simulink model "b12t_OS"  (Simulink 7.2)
settings: Solver=ode3  SolverMode=SingleTasking  StartTime=0.0  StopTime=0.2  FixedStep=10e-6  MaxStep=1e-5  RelTol=1e-4  AbsTol=1e-4

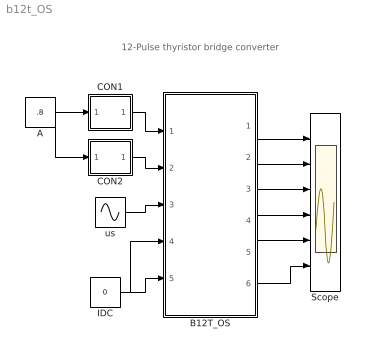
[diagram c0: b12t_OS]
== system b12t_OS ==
  note: 12-Pulse thyristor bridge converter
  A : Constant  Value=.8
  B12T_OS : Subsystem  mask{LS=1e-4, LT1=1e-4, LT2=1e-4, LD=1e-3, ILD0=200, C=5e-3, VC0=500, RL=2}
      mask prompts: LS "source Inductance"; LT1 "TYY leakage Inductance"; LT2 "TYD leakage Inductance"; LD "DC Inductance"; ILD0 "Initial Current ILD0"; C "Load Capacitance"; VC0 "Initial Cap Voltage"; RL "Load Resistance"
      mask help: 12-Pulse Thyristor Bridge Converter Input Vector u: u[0]= B6T1_H1.gate u[1]= B6T1_H2.gate u[2]= B6T1_H3.gate u[3]= B6T1_H4.gate u[4]= B6T1_H5.gate u[5]= B6T1_H6.gate u[6]= B6T2_H1.gate u[7]= B6T2_H2.gate u[8]= B6T2_H3.gate u[9]= B6T2_H4.gate u[10]= B6T2_H5.gate u[11]= B6T2_H6.gate u[12]= Vs1.v u[13]= Vs2.v u[14]= Vs3.v u[15]= IDC1.i u[16]= IDC1.i Output Vector y: y[0]= B6T1_T11.I y[1]= B6T1_T11.V y[2]= B6T2_T11.I y[3]= B6T2_T11.V y[4]= Ls1.I y[5]= Ls2.I y[6]= Ls3.I y[7]= Ld1.I y[8]= Ld2.I y[6]= VDC.V y[9]= VC1.V y[10]= VC2.V Parameter Vector p: p[0]= Ls.L p[1]= TYY_LT.L p[2]= TYD_LT.L p[3]= Ld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
  CON1 : Subsystem  mask(B6THY-Con){F=50, PH=60, TD=2e-3}
      mask prompts: F "Frequency"; PH "Phase Angle (Degree)"; TD "Puls Duration"
      mask help: Control of one Thyristor in a line commutated Converter circuit
      mask init:
      | x=0:pi/20:2*pi;
      | y=cos(x);
  CON2 : Subsystem  mask(B6THY-Con){F=50, PH=-150+60, TD=2e-3}
      mask prompts: F "Frequency"; PH "Phase Angle (Degree)"; TD "Puls Duration"
      mask help: Control of one Thyristor in a line commutated Converter circuit
      mask init:
      | x=0:pi/20:2*pi;
      | y=cos(x);
  IDC : Constant  Value=0
  Scope : Scope  NumInputPorts=6
  us : Sin  Amplitude=230*sqrt(2)  Frequency=2*pi*50  Phase="[0,  -2*pi/3,  -4*pi/3]"  SampleTime=0
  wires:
  A/1 -> CON1/1(In1), CON2/1(In1)
  CON1/1(Out1) -> B12T_OS/1(SWs)
  us/1 -> B12T_OS/3(vS)
  CON2/1(Out1) -> B12T_OS/2(SWs1)
  B12T_OS/1(i1T1;v1T!) -> Scope/1
  B12T_OS/2(i2T1,i2T1) -> Scope/2
  B12T_OS/3("iL1, iL2, iL3") -> Scope/3
  IDC/1 -> B12T_OS/4(iDC1), B12T_OS/5(iDC2)
  B12T_OS/4(iDC1,iDC2) -> Scope/4
  B12T_OS/5(vDC1,vDC1) -> Scope/5
  B12T_OS/6(vC1,vC2) -> Scope/6

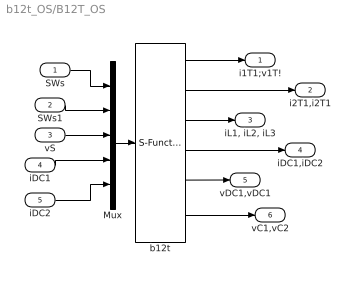
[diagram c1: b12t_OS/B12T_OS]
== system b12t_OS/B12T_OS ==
  SWs : Inport  OutDataType=sfix(16)  OutScaling=2^0
  SWs1 : Inport  Port=2  OutDataType=sfix(16)  OutScaling=2^0
  vS : Inport  Port=3  OutDataType=sfix(16)  OutScaling=2^0
  iDC1 : Inport  Port=4  OutDataType=sfix(16)  OutScaling=2^0
  iDC2 : Inport  Port=5  OutDataType=sfix(16)  OutScaling=2^0
  Mux : Mux  Inputs="[6   6   3  1  1]"
  b12t : S-Function  FunctionName=s_b12t_OS  Parameters="[LS  LT1 LT2  LD ILD0  C  VC0 RL]"  EnableBusSupport=off
  i1T1;v1T! : Outport  OutDataType=sfix(16)  OutScaling=2^0
  i2T1,i2T1 : Outport  Port=2  OutDataType=sfix(16)  OutScaling=2^0
  "iL1, iL2, iL3" : Outport  Port=3  OutDataType=sfix(16)  OutScaling=2^0
  iDC1,iDC2 : Outport  Port=4  OutDataType=sfix(16)  OutScaling=2^0
  vDC1,vDC1 : Outport  Port=5  OutDataType=sfix(16)  OutScaling=2^0
  vC1,vC2 : Outport  Port=6  OutDataType=sfix(16)  OutScaling=2^0
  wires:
  Mux/1 -> b12t/1
  iDC1/1 -> Mux/4
  b12t/2 -> i2T1,i2T1/1
  b12t/1 -> i1T1;v1T!/1
  vS/1 -> Mux/3
  SWs/1 -> Mux/1
  SWs1/1 -> Mux/2
  iDC2/1 -> Mux/5
  b12t/3 -> "iL1, iL2, iL3"/1
  b12t/4 -> iDC1,iDC2/1
  b12t/5 -> vDC1,vDC1/1
  b12t/6 -> vC1,vC2/1

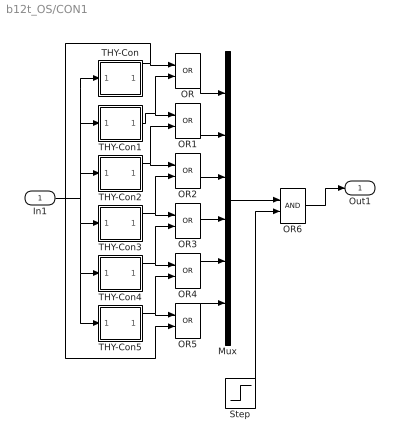
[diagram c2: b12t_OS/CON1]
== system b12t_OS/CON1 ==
  In1 : Inport
  Mux : Mux  Inputs=6
  OR{,1..5} (6 alike) : Logic  Operator=OR
  OR6 : Logic
  Step : Step  Time=1e-4  SampleTime=0
  THY-Con : Subsystem  mask(THY-Con){F=F, PH=PH, TD=TD}
      mask prompts: F "Frequency"; PH "Phase Angle (Degree)"; TD "Puls Duration"
      mask init:
      | x=0:pi/20:2*pi;
      | y=cos(x);
  THY-Con1 : Subsystem  mask(THY-Con){F=F, PH=PH-60, TD=TD}
      mask prompts: F "Frequency"; PH "Phase Angle (Degree)"; TD "Puls Duration"
      mask init:
      | x=0:pi/20:2*pi;
      | y=cos(x);
  THY-Con2 : Subsystem  mask(THY-Con){F=F, PH=PH-120, TD=TD}
      mask prompts: F "Frequency"; PH "Phase Angle (Degree)"; TD "Puls Duration"
      mask init:
      | x=0:pi/20:2*pi;
      | y=cos(x);
  THY-Con3 : Subsystem  mask(THY-Con){F=F, PH=PH-180, TD=TD}
      mask prompts: F "Frequency"; PH "Phase Angle (Degree)"; TD "Puls Duration"
      mask init:
      | x=0:pi/20:2*pi;
      | y=cos(x);
  THY-Con4 : Subsystem  mask(THY-Con){F=F, PH=PH-240, TD=TD}
      mask prompts: F "Frequency"; PH "Phase Angle (Degree)"; TD "Puls Duration"
      mask init:
      | x=0:pi/20:2*pi;
      | y=cos(x);
  THY-Con5 : Subsystem  mask(THY-Con){F=F, PH=PH-300, TD=TD}
      mask prompts: F "Frequency"; PH "Phase Angle (Degree)"; TD "Puls Duration"
      mask init:
      | x=0:pi/20:2*pi;
      | y=cos(x);
  Out1 : Outport
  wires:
  Step/1 -> OR6/2
  Mux/1 -> OR6/1
  In1/1 -> THY-Con/1(In1), THY-Con1/1(In1), THY-Con2/1(In1), THY-Con3/1(In1), THY-Con4/1(In1), THY-Con5/1(In1)
  THY-Con1/1(Out1) -> OR1/1, OR/2
  THY-Con2/1(Out1) -> OR2/1, OR1/2
  THY-Con3/1(Out1) -> OR3/1, OR2/2
  THY-Con4/1(Out1) -> OR4/1, OR3/2
  THY-Con5/1(Out1) -> OR5/1, OR4/2
  THY-Con/1(Out1) -> OR/1, OR5/2
  OR/1 -> Mux/1
  OR1/1 -> Mux/2
  OR2/1 -> Mux/3
  OR3/1 -> Mux/4
  OR4/1 -> Mux/5
  OR5/1 -> Mux/6
  OR6/1 -> Out1/1

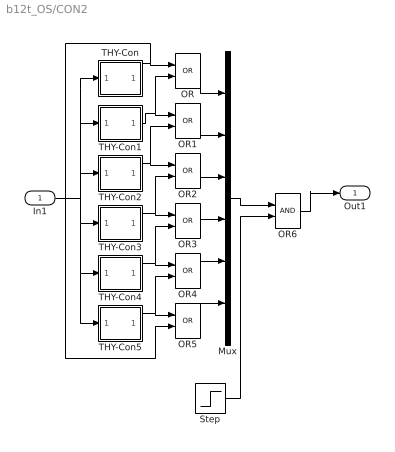
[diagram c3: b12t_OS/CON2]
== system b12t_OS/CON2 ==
  In1 : Inport
  Mux : Mux  Inputs=6
  OR{,1..5} (6 alike) : Logic  Operator=OR
  OR6 : Logic
  Step : Step  Time=1e-4  SampleTime=0
  THY-Con : Subsystem  mask(THY-Con){F=F, PH=PH, TD=TD}
      mask prompts: F "Frequency"; PH "Phase Angle (Degree)"; TD "Puls Duration"
      mask init:
      | x=0:pi/20:2*pi;
      | y=cos(x);
  THY-Con1 : Subsystem  mask(THY-Con){F=F, PH=PH-60, TD=TD}
      mask prompts: F "Frequency"; PH "Phase Angle (Degree)"; TD "Puls Duration"
      mask init:
      | x=0:pi/20:2*pi;
      | y=cos(x);
  THY-Con2 : Subsystem  mask(THY-Con){F=F, PH=PH-120, TD=TD}
      mask prompts: F "Frequency"; PH "Phase Angle (Degree)"; TD "Puls Duration"
      mask init:
      | x=0:pi/20:2*pi;
      | y=cos(x);
  THY-Con3 : Subsystem  mask(THY-Con){F=F, PH=PH-180, TD=TD}
      mask prompts: F "Frequency"; PH "Phase Angle (Degree)"; TD "Puls Duration"
      mask init:
      | x=0:pi/20:2*pi;
      | y=cos(x);
  THY-Con4 : Subsystem  mask(THY-Con){F=F, PH=PH-240, TD=TD}
      mask prompts: F "Frequency"; PH "Phase Angle (Degree)"; TD "Puls Duration"
      mask init:
      | x=0:pi/20:2*pi;
      | y=cos(x);
  THY-Con5 : Subsystem  mask(THY-Con){F=F, PH=PH-300, TD=TD}
      mask prompts: F "Frequency"; PH "Phase Angle (Degree)"; TD "Puls Duration"
      mask init:
      | x=0:pi/20:2*pi;
      | y=cos(x);
  Out1 : Outport
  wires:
  Step/1 -> OR6/2
  In1/1 -> THY-Con/1(In1), THY-Con1/1(In1), THY-Con2/1(In1), THY-Con3/1(In1), THY-Con4/1(In1), THY-Con5/1(In1)
  THY-Con1/1(Out1) -> OR1/1, OR/2
  THY-Con2/1(Out1) -> OR2/1, OR1/2
  THY-Con3/1(Out1) -> OR3/1, OR2/2
  THY-Con4/1(Out1) -> OR4/1, OR3/2
  THY-Con5/1(Out1) -> OR5/1, OR4/2
  THY-Con/1(Out1) -> OR/1, OR5/2
  OR/1 -> Mux/1
  OR1/1 -> Mux/2
  OR2/1 -> Mux/3
  OR3/1 -> Mux/4
  OR4/1 -> Mux/5
  OR5/1 -> Mux/6
  Mux/1 -> OR6/1
  OR6/1 -> Out1/1

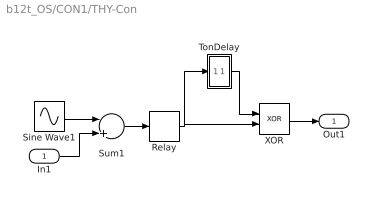
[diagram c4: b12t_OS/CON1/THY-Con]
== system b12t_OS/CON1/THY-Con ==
  In1 : Inport
  Relay : Relay
  Sine Wave1 : Sin  Frequency=F*2*pi  Phase=PH*pi/180  SampleTime=0
  Sum1 : Sum  Inputs=-+
  TonDelay : Subsystem  mask(TonDelay){DT=TD}
      mask prompts: DT "Dead Time"
      mask help: Turn on dead time to protect against short circuit of the converter leg
  XOR : Logic  Operator=XOR
  Out1 : Outport
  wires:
  In1/1 -> Sum1/2
  Sum1/1 -> Relay/1
  TonDelay/1(s1d) -> XOR/1
  Relay/1 -> TonDelay/1(s1), XOR/2
  XOR/1 -> Out1/1
  Sine Wave1/1 -> Sum1/1

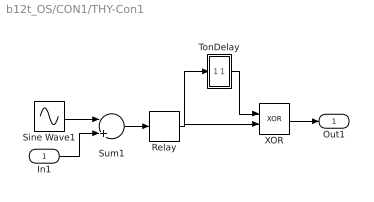
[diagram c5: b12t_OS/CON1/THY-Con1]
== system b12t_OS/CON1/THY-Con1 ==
  In1 : Inport
  Relay : Relay
  Sine Wave1 : Sin  Frequency=F*2*pi  Phase=PH*pi/180  SampleTime=0
  Sum1 : Sum  Inputs=-+
  TonDelay : Subsystem  mask(TonDelay){DT=TD}
      mask prompts: DT "Dead Time"
      mask help: Turn on dead time to protect against short circuit of the converter leg
  XOR : Logic  Operator=XOR
  Out1 : Outport
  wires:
  In1/1 -> Sum1/2
  Sum1/1 -> Relay/1
  TonDelay/1(s1d) -> XOR/1
  Relay/1 -> TonDelay/1(s1), XOR/2
  XOR/1 -> Out1/1
  Sine Wave1/1 -> Sum1/1

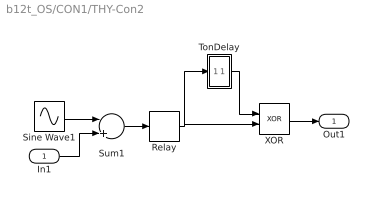
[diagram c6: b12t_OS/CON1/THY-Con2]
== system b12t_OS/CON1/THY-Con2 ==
  In1 : Inport
  Relay : Relay
  Sine Wave1 : Sin  Frequency=F*2*pi  Phase=PH*pi/180  SampleTime=0
  Sum1 : Sum  Inputs=-+
  TonDelay : Subsystem  mask(TonDelay){DT=TD}
      mask prompts: DT "Dead Time"
      mask help: Turn on dead time to protect against short circuit of the converter leg
  XOR : Logic  Operator=XOR
  Out1 : Outport
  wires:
  In1/1 -> Sum1/2
  Sum1/1 -> Relay/1
  TonDelay/1(s1d) -> XOR/1
  Relay/1 -> TonDelay/1(s1), XOR/2
  XOR/1 -> Out1/1
  Sine Wave1/1 -> Sum1/1

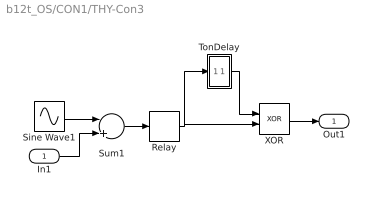
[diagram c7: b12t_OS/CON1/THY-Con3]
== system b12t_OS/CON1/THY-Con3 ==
  In1 : Inport
  Relay : Relay
  Sine Wave1 : Sin  Frequency=F*2*pi  Phase=PH*pi/180  SampleTime=0
  Sum1 : Sum  Inputs=-+
  TonDelay : Subsystem  mask(TonDelay){DT=TD}
      mask prompts: DT "Dead Time"
      mask help: Turn on dead time to protect against short circuit of the converter leg
  XOR : Logic  Operator=XOR
  Out1 : Outport
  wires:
  In1/1 -> Sum1/2
  Sum1/1 -> Relay/1
  TonDelay/1(s1d) -> XOR/1
  Relay/1 -> TonDelay/1(s1), XOR/2
  XOR/1 -> Out1/1
  Sine Wave1/1 -> Sum1/1

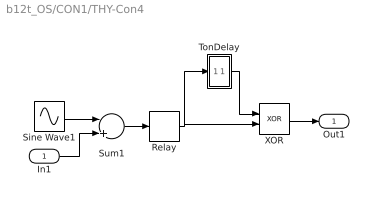
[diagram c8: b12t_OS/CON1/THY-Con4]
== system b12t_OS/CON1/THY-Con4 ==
  In1 : Inport
  Relay : Relay
  Sine Wave1 : Sin  Frequency=F*2*pi  Phase=PH*pi/180  SampleTime=0
  Sum1 : Sum  Inputs=-+
  TonDelay : Subsystem  mask(TonDelay){DT=TD}
      mask prompts: DT "Dead Time"
      mask help: Turn on dead time to protect against short circuit of the converter leg
  XOR : Logic  Operator=XOR
  Out1 : Outport
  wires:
  In1/1 -> Sum1/2
  Sum1/1 -> Relay/1
  TonDelay/1(s1d) -> XOR/1
  Relay/1 -> TonDelay/1(s1), XOR/2
  XOR/1 -> Out1/1
  Sine Wave1/1 -> Sum1/1

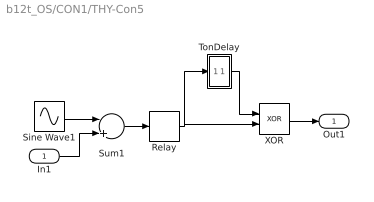
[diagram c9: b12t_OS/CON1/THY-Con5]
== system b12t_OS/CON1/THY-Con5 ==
  In1 : Inport
  Relay : Relay
  Sine Wave1 : Sin  Frequency=F*2*pi  Phase=PH*pi/180  SampleTime=0
  Sum1 : Sum  Inputs=-+
  TonDelay : Subsystem  mask(TonDelay){DT=TD}
      mask prompts: DT "Dead Time"
      mask help: Turn on dead time to protect against short circuit of the converter leg
  XOR : Logic  Operator=XOR
  Out1 : Outport
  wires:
  In1/1 -> Sum1/2
  Sum1/1 -> Relay/1
  TonDelay/1(s1d) -> XOR/1
  Relay/1 -> TonDelay/1(s1), XOR/2
  XOR/1 -> Out1/1
  Sine Wave1/1 -> Sum1/1

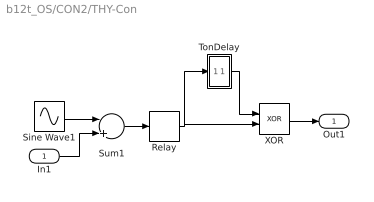
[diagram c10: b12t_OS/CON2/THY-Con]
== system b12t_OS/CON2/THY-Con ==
  In1 : Inport
  Relay : Relay
  Sine Wave1 : Sin  Frequency=F*2*pi  Phase=PH*pi/180  SampleTime=0
  Sum1 : Sum  Inputs=-+
  TonDelay : Subsystem  mask(TonDelay){DT=TD}
      mask prompts: DT "Dead Time"
      mask help: Turn on dead time to protect against short circuit of the converter leg
  XOR : Logic  Operator=XOR
  Out1 : Outport
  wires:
  In1/1 -> Sum1/2
  Sum1/1 -> Relay/1
  TonDelay/1(s1d) -> XOR/1
  Relay/1 -> TonDelay/1(s1), XOR/2
  XOR/1 -> Out1/1
  Sine Wave1/1 -> Sum1/1

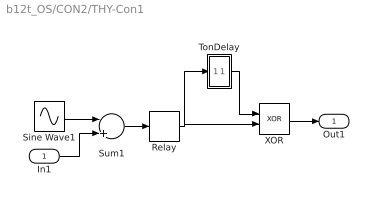
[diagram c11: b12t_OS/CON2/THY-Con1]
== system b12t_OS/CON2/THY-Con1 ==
  In1 : Inport
  Relay : Relay
  Sine Wave1 : Sin  Frequency=F*2*pi  Phase=PH*pi/180  SampleTime=0
  Sum1 : Sum  Inputs=-+
  TonDelay : Subsystem  mask(TonDelay){DT=TD}
      mask prompts: DT "Dead Time"
      mask help: Turn on dead time to protect against short circuit of the converter leg
  XOR : Logic  Operator=XOR
  Out1 : Outport
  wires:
  In1/1 -> Sum1/2
  Sum1/1 -> Relay/1
  TonDelay/1(s1d) -> XOR/1
  Relay/1 -> TonDelay/1(s1), XOR/2
  XOR/1 -> Out1/1
  Sine Wave1/1 -> Sum1/1

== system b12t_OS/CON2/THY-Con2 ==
  In1 : Inport
  Relay : Relay
  Sine Wave1 : Sin  Frequency=F*2*pi  Phase=PH*pi/180  SampleTime=0
  Sum1 : Sum  Inputs=-+
  TonDelay : Subsystem  mask(TonDelay){DT=TD}
      mask prompts: DT "Dead Time"
      mask help: Turn on dead time to protect against short circuit of the converter leg
  XOR : Logic  Operator=XOR
  Out1 : Outport
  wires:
  In1/1 -> Sum1/2
  Sum1/1 -> Relay/1
  TonDelay/1(s1d) -> XOR/1
  Relay/1 -> TonDelay/1(s1), XOR/2
  XOR/1 -> Out1/1
  Sine Wave1/1 -> Sum1/1

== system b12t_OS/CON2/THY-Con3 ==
  In1 : Inport
  Relay : Relay
  Sine Wave1 : Sin  Frequency=F*2*pi  Phase=PH*pi/180  SampleTime=0
  Sum1 : Sum  Inputs=-+
  TonDelay : Subsystem  mask(TonDelay){DT=TD}
      mask prompts: DT "Dead Time"
      mask help: Turn on dead time to protect against short circuit of the converter leg
  XOR : Logic  Operator=XOR
  Out1 : Outport
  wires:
  In1/1 -> Sum1/2
  Sum1/1 -> Relay/1
  TonDelay/1(s1d) -> XOR/1
  Relay/1 -> TonDelay/1(s1), XOR/2
  XOR/1 -> Out1/1
  Sine Wave1/1 -> Sum1/1

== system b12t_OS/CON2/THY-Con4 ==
  In1 : Inport
  Relay : Relay
  Sine Wave1 : Sin  Frequency=F*2*pi  Phase=PH*pi/180  SampleTime=0
  Sum1 : Sum  Inputs=-+
  TonDelay : Subsystem  mask(TonDelay){DT=TD}
      mask prompts: DT "Dead Time"
      mask help: Turn on dead time to protect against short circuit of the converter leg
  XOR : Logic  Operator=XOR
  Out1 : Outport
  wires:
  In1/1 -> Sum1/2
  Sum1/1 -> Relay/1
  TonDelay/1(s1d) -> XOR/1
  Relay/1 -> TonDelay/1(s1), XOR/2
  XOR/1 -> Out1/1
  Sine Wave1/1 -> Sum1/1

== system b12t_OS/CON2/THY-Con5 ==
  In1 : Inport
  Relay : Relay
  Sine Wave1 : Sin  Frequency=F*2*pi  Phase=PH*pi/180  SampleTime=0
  Sum1 : Sum  Inputs=-+
  TonDelay : Subsystem  mask(TonDelay){DT=TD}
      mask prompts: DT "Dead Time"
      mask help: Turn on dead time to protect against short circuit of the converter leg
  XOR : Logic  Operator=XOR
  Out1 : Outport
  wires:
  In1/1 -> Sum1/2
  Sum1/1 -> Relay/1
  TonDelay/1(s1d) -> XOR/1
  Relay/1 -> TonDelay/1(s1), XOR/2
  XOR/1 -> Out1/1
  Sine Wave1/1 -> Sum1/1

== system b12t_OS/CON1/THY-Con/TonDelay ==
  s1 : Inport
  Int : Integrator  ExternalReset=falling
  Rel1 : Relay  OnSwitchValue=DT
  s1d : Outport  InitialOutput=0
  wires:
  Int/1 -> Rel1/1
  s1/1 -> Int/2, Int/1
  Rel1/1 -> s1d/1

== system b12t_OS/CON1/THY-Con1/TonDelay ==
  s1 : Inport
  Int : Integrator  ExternalReset=falling
  Rel1 : Relay  OnSwitchValue=DT
  s1d : Outport  InitialOutput=0
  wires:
  Int/1 -> Rel1/1
  s1/1 -> Int/2, Int/1
  Rel1/1 -> s1d/1

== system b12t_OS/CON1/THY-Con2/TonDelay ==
  s1 : Inport
  Int : Integrator  ExternalReset=falling
  Rel1 : Relay  OnSwitchValue=DT
  s1d : Outport  InitialOutput=0
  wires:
  Int/1 -> Rel1/1
  s1/1 -> Int/2, Int/1
  Rel1/1 -> s1d/1

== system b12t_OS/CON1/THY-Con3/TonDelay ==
  s1 : Inport
  Int : Integrator  ExternalReset=falling
  Rel1 : Relay  OnSwitchValue=DT
  s1d : Outport  InitialOutput=0
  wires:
  Int/1 -> Rel1/1
  s1/1 -> Int/2, Int/1
  Rel1/1 -> s1d/1

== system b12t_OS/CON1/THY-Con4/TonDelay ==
  s1 : Inport
  Int : Integrator  ExternalReset=falling
  Rel1 : Relay  OnSwitchValue=DT
  s1d : Outport  InitialOutput=0
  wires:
  Int/1 -> Rel1/1
  s1/1 -> Int/2, Int/1
  Rel1/1 -> s1d/1

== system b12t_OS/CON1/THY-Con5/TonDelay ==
  s1 : Inport
  Int : Integrator  ExternalReset=falling
  Rel1 : Relay  OnSwitchValue=DT
  s1d : Outport  InitialOutput=0
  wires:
  Int/1 -> Rel1/1
  s1/1 -> Int/2, Int/1
  Rel1/1 -> s1d/1

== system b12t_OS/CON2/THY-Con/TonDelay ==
  s1 : Inport
  Int : Integrator  ExternalReset=falling
  Rel1 : Relay  OnSwitchValue=DT
  s1d : Outport  InitialOutput=0
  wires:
  Int/1 -> Rel1/1
  s1/1 -> Int/2, Int/1
  Rel1/1 -> s1d/1

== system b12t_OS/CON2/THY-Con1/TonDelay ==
  s1 : Inport
  Int : Integrator  ExternalReset=falling
  Rel1 : Relay  OnSwitchValue=DT
  s1d : Outport  InitialOutput=0
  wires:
  Int/1 -> Rel1/1
  s1/1 -> Int/2, Int/1
  Rel1/1 -> s1d/1

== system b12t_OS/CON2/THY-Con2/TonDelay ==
  s1 : Inport
  Int : Integrator  ExternalReset=falling
  Rel1 : Relay  OnSwitchValue=DT
  s1d : Outport  InitialOutput=0
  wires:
  Int/1 -> Rel1/1
  s1/1 -> Int/2, Int/1
  Rel1/1 -> s1d/1

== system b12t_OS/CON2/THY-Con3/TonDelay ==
  s1 : Inport
  Int : Integrator  ExternalReset=falling
  Rel1 : Relay  OnSwitchValue=DT
  s1d : Outport  InitialOutput=0
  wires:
  Int/1 -> Rel1/1
  s1/1 -> Int/2, Int/1
  Rel1/1 -> s1d/1

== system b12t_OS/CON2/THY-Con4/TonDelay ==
  s1 : Inport
  Int : Integrator  ExternalReset=falling
  Rel1 : Relay  OnSwitchValue=DT
  s1d : Outport  InitialOutput=0
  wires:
  Int/1 -> Rel1/1
  s1/1 -> Int/2, Int/1
  Rel1/1 -> s1d/1

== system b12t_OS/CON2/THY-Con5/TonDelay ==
  s1 : Inport
  Int : Integrator  ExternalReset=falling
  Rel1 : Relay  OnSwitchValue=DT
  s1d : Outport  InitialOutput=0
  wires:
  Int/1 -> Rel1/1
  s1/1 -> Int/2, Int/1
  Rel1/1 -> s1d/1
